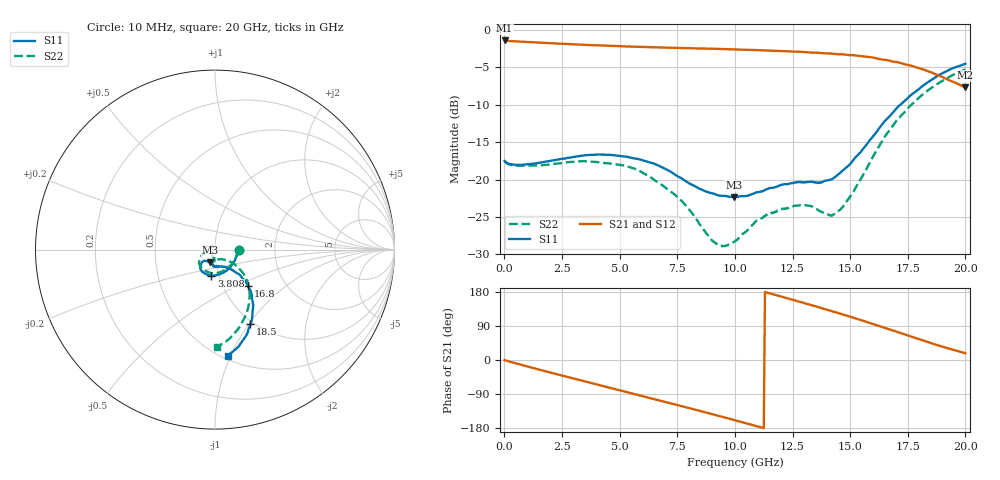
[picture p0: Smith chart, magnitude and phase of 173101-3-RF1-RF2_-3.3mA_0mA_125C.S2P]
!  2-Port S-parameters saved by WinCal
! VAR MeasName=S-Parameters (CALIBRATED_DATA) read from VNA (N5242A)
! VAR MeasDate=2017-7-20 10:58:00
! VAR NAME=173101-3-RF1-RF2_-3.3mA_0mA_125C
! VAR FILENAME=173101-3-RF1-RF2_-3.3mA_0mA_125C.S2P
! VAR DATE=2017-7-20 10:58:00
! VAR PHYS_PORTS=1,2
# Hz S DB R 50
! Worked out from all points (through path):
!   401 points, 10 MHz to 20 GHz, reference 50 ohm
!   highest |S21| = -1.39 dB at 10 MHz (marker M1); lowest = -7.7 dB at 20 GHz (marker M2)
!   group delay of S21, straight-line fit = 47 ps
!   lowest |S11| = -22.3 dB at 9.955 GHz (marker M3), VSWR 1.17, Z = 46.8 - j6.67 ohm
!   |S11| at or under -10 dB: start of sweep to 17.17 GHz
!   |S22| runs from -28.9 to -5.3 dB; largest |S21 - S12| = 0.0041
!   S11 on the Smith chart (normalised r, x): 10 MHz: 1.31, -0.01; 3.808 GHz: 0.92, -0.27; 16.8 GHz: 1.31, -0.58; 18.5 GHz: 0.96, -1.02; 20 GHz: 0.53, -0.98
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1e7  -17.53 -1.1  -1.39 -0.2  -1.40 -0.2  -17.54 -0.9
1.559225e9  -17.74 -49.7  -1.69 -26.2  -1.69 -26.2  -18.11 -51.7
3.358325e9  -16.82 -90.4  -1.97 -54.5  -1.97 -54.5  -17.54 -96.8
3.8081e9  -16.71 -97.7  -2.02 -61.4  -2.02 -61.5  -17.62 -105.8
5.2074e9  -16.91 -118.6  -2.19 -83.1  -2.20 -83.1  -18.12 -131.3
6.70665e9  -18.17 -131.1  -2.32 -106.4  -2.31 -106.3  -20.48 -151.2
7.756125e9  -19.98 -135.6  -2.41 -122.8  -2.42 -122.8  -23.08 -159.8
9.10545e9  -21.91 -126.4  -2.50 -144.3  -2.50 -144.4  -28.36 -144.4
9.455275e9  -22.18 -120.6  -2.55 -150.1  -2.54 -150.1  -28.92 -131.1
9.955025e9  -22.34 -111.8  -2.59 -158.2  -2.59 -158.3  -28.35 -112.8
1.0005e10  -22.30 -111.5  -2.60 -159.0  -2.60 -159.1  -28.26 -111.4
1.095452e10  -21.70 -100.6  -2.68 -174.6  -2.69 -174.7  -25.47 -92.9
1.165418e10  -21.11 -96.8  -2.76 173.6  -2.76 173.5  -24.41 -93.0
1.335332e10  -20.28 -83.5  -3.01 144.2  -2.99 144.3  -23.62 -93.1
1.415292e10  -20.01 -68.8  -3.13 129.9  -3.14 129.8  -24.79 -71.4
1.46027e10  -19.00 -60.5  -3.24 121.6  -3.24 121.7  -23.93 -56.1
1.575212e10  -15.17 -47.4  -3.59 99.4  -3.58 99.4  -18.34 -37.2
1.670165e10  -11.56 -47.1  -4.08 80.8  -4.12 80.5  -13.41 -40.8
1.68016e10  -11.23 -47.9  -4.19 78.8  -4.18 79.1  -13.00 -42.0
1.775112e10  -8.44 -56.0  -4.88 59.6  -4.88 59.7  -9.73 -53.8
1.850075e10  -6.74 -64.7  -5.65 44.7  -5.68 44.6  -7.80 -65.6
2e10  -4.51 -83.1  -7.68 17.9  -7.72 18.3  -5.29 -89.0
